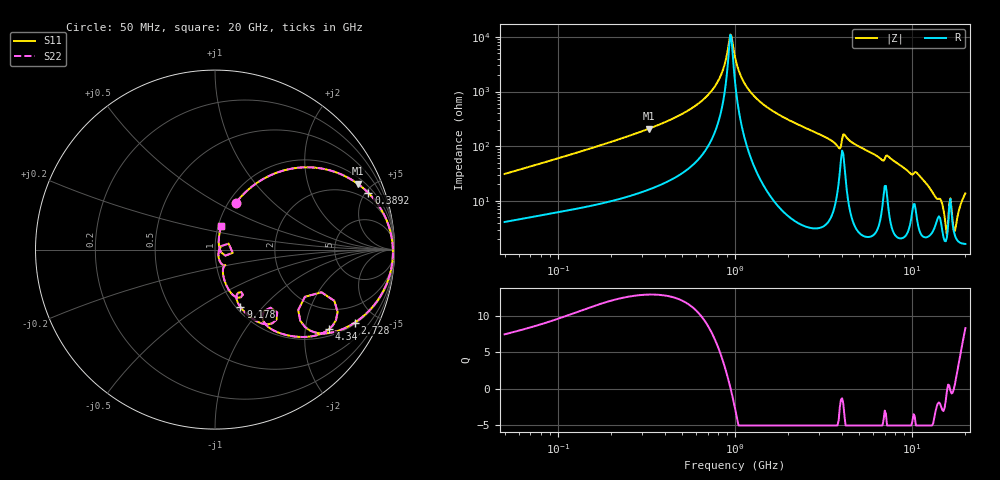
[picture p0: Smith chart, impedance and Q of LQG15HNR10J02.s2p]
!Murata Part Number: LQG15HNR10J02
!These Parameters are Measured in Series Mode Connection
!  o--[Z]--o
!Port1  Port2
!  o-------o
!Freq. Start=50[MHz] Stop=20[GHz], 401[Steps]
# Hz S RI R 50
!Freq.(Hz) S11(Real) S11(Imag) S21(Real) S21(Imag) S12(Real) S12(Imag) S22(Real) S22(Imag)
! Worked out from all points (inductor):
!   401 points, 50 MHz to 20 GHz, reference 50 ohm
!   read as one part in series: L = 96.3 nH near 51.52 MHz
!   highest Q = 12.9 at 325.2 MHz (marker M1), where L = 102 nH
!   self-resonance near 941.8 MHz
!   S11 on the Smith chart (normalised r, x): 50 MHz: 1.08, +0.62; 389.2 MHz: 1.41, +5.24; 2.728 GHz: 1.06, -3.80; 4.34 GHz: 1.22, -2.70; 9.178 GHz: 1.05, -0.76; 20 GHz: 1.03, +0.27
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5e7  0.1171 0.2616  0.8829 -0.2616  0.8829 -0.2616  0.1171 0.2616
1.364002e8  0.4065 0.447  0.5935 -0.447  0.5935 -0.447  0.4065 0.447
3.251725e8  0.7946 0.3672  0.2054 -0.3672  0.2054 -0.3672  0.7946 0.3672
3.721004e8  0.841 0.329  0.159 -0.329  0.159 -0.329  0.841 0.329
3.892024e8  0.855 0.3153  0.145 -0.3153  0.145 -0.3153  0.855 0.3153
7.30116e8  0.9778 0.0971  0.0222 -0.0971  0.0222 -0.0971  0.9778 0.0971
8.354841e8  0.9874 0.0468  0.0126 -0.0468  0.0126 -0.0468  0.9874 0.0468
9.418449e8  0.9911 0.00143  0.00888 -0.00143  0.00888 -0.00143  0.9911 0.00143
1e9  0.9913 -0.0215  0.00869 0.0215  0.00869 0.0215  0.9913 -0.0215
1.110545e9  0.9889 -0.0619  0.0111 0.0619  0.0111 0.0619  0.9889 -0.0619
1.329223e9  0.976 -0.1321  0.024 0.1321  0.024 0.1321  0.976 -0.1321
2.728004e9  0.7796 -0.4063  0.2204 0.4063  0.2204 0.4063  0.7796 -0.4063
3.850025e9  0.4749 -0.3962  0.5251 0.3962  0.5251 0.3962  0.4749 -0.3962
4.34015e9  0.637 -0.4421  0.363 0.4421  0.363 0.4421  0.637 -0.4421
7.442007e9  0.2972 -0.4161  0.7028 0.4161  0.7028 0.4161  0.2972 -0.4161
9.178299e9  0.1417 -0.32  0.8583 0.32  0.8583 0.32  0.1417 -0.32
1.098561e10  0.0993 -0.2528  0.9007 0.2528  0.9007 0.2528  0.0993 -0.2528
1.438523e10  0.0547 -0.0883  0.9453 0.0883  0.9453 0.0883  0.0547 -0.0883
1.550395e10  0.0187 -0.0268  0.9813 0.0268  0.9813 0.0268  0.0187 -0.0268
1.646126e10  0.0986 -0.018  0.9014 0.018  0.9014 0.018  0.0986 -0.018
1.747767e10  0.0228 0.0161  0.9772 -0.0161  0.9772 -0.0161  0.0228 0.0161
2e10  0.0335 0.1297  0.9665 -0.1297  0.9665 -0.1297  0.0335 0.1297
